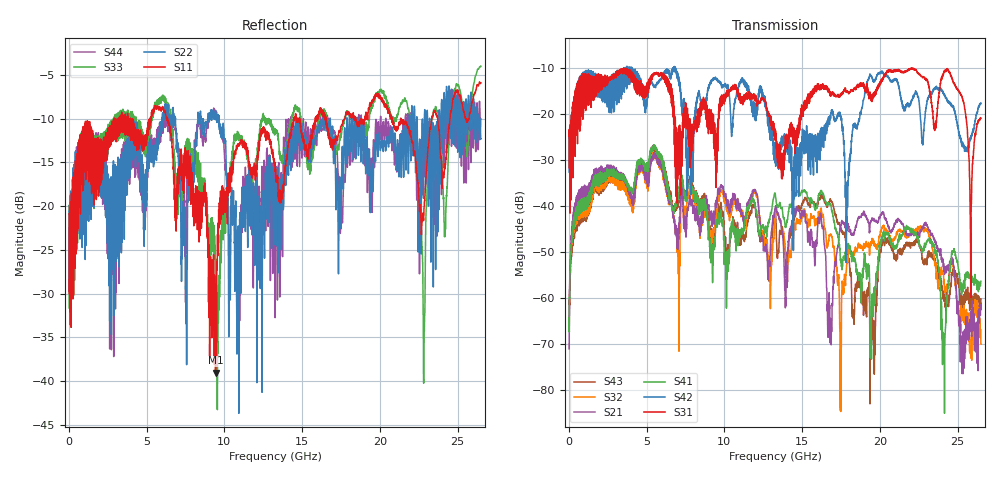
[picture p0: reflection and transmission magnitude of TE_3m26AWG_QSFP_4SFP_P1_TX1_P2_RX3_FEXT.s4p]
!Agilent Technologies,N5222A,MY51421691,A.10.00.00
!Agilent N5222A: A.10.00.00
!Date: Friday, January 30, 2015 12:37:53
!Correction: S11(Full 4 Port(1,2,3,4))
!S12(Full 4 Port(1,2,3,4))
!S13(Full 4 Port(1,2,3,4))
!S14(Full 4 Port(1,2,3,4))
!S21(Full 4 Port(1,2,3,4))
!S22(Full 4 Port(1,2,3,4))
!S23(Full 4 Port(1,2,3,4))
!S24(Full 4 Port(1,2,3,4))
!S31(Full 4 Port(1,2,3,4))
!S32(Full 4 Port(1,2,3,4))
!S33(Full 4 Port(1,2,3,4))
!S34(Full 4 Port(1,2,3,4))
!S41(Full 4 Port(1,2,3,4))
!S42(Full 4 Port(1,2,3,4))
!S43(Full 4 Port(1,2,3,4))
!S44(Full 4 Port(1,2,3,4))
!S4P File: Measurements: <S11,S12,S13,S14>,
!<S21,S22,S23,S24>,
!<S31,S32,S33,S34>,
!<S41,S42,S43,S44>:
# Hz S  dB  R 50.0
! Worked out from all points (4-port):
!   2650 points, 10 MHz to 26.5 GHz, reference 50 ohm
!   strongest paths, dB at 10 MHz, 6.63 GHz, 13.26 GHz, 19.88 GHz, 26.5 GHz:
!     S31: -24.7, -18.2, -24.4, -13.6, -20.8
!     S42: -25.1, -10.6, -28.6, -11.1, -17.5
!     S41: -64.3, -40.3, -37.2, -52.6, -56.3
!     S21: -71.0, -39.8, -40.4, -43.5, -61.4
!     S32: -66.2, -39.8, -42.4, -48.5, -70.0
!     S43: -66.0, -39.3, -41.0, -54.0, -60.1
!   lowest |S11| = -39.0 dB at 9.43 GHz (marker M1), VSWR 1.02, Z = 50.5 + j1.01 ohm
!   |S11| at or under -10 dB: start of sweep to 2.939 GHz; 6.342 GHz to 14.45 GHz (8.109 GHz wide, 78 % of centre); 21.35 GHz to 23.33 GHz (1.977 GHz wide, 8.85 % of centre)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
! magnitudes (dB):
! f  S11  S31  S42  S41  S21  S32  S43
! 10 MHz  -20.9  -24.7  -25.1  -64.3  -71.0  -66.2  -66.0
! 1.74 GHz  -12.3  -11.4  -11.3  -35.2  -34.1  -36.0  -36.6
! 9.43 GHz  -39.0  -27.3  -12.3  -45.1  -39.7  -42.6  -43.8
! 17.87 GHz  -9.3  -14.9  -43.5  -49.9  -44.6  -52.7  -48.6
! 19.35 GHz  -8.4  -15.2  -11.4  -57.7  -45.5  -50.3  -66.0
! 22.81 GHz  -21.7  -11.8  -23.8  -49.6  -44.8  -45.5  -51.8
! 26.5 GHz  -5.9  -20.8  -17.5  -56.3  -61.4  -70.0  -60.1
